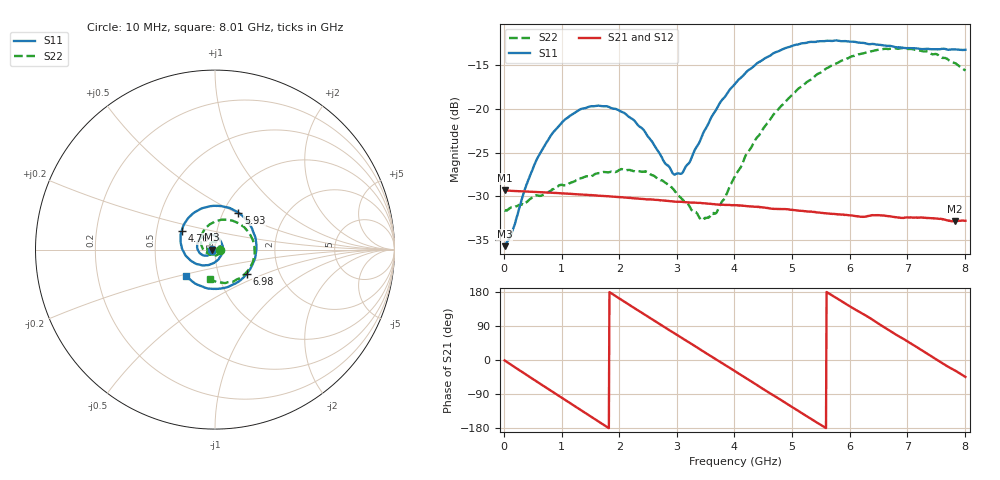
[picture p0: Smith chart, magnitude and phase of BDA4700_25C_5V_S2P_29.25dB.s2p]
!Agilent Technologies,E5071B,MY42404982,A.09.10
!Date: Mon Oct 20 13:41:18 2025
!Data & Calibration Information:
!Freq	S11:SOLT2(ON)	S21:SOLT2(ON)	S12:SOLT2(ON)	S22:SOLT2(ON)
# Hz S RI R 50
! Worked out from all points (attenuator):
!   801 points, 10 MHz to 8.01 GHz, reference 50 ohm
!   highest |S21| = -29.31 dB at 10 MHz (marker M1); lowest = -32.9 dB at 7.83 GHz (marker M2)
!   lowest |S11| = -35.7 dB at 10 MHz (marker M3), VSWR 1.03, Z = 48.4 - j0.111 ohm
!   |S11| at or under -10 dB: start of sweep to end of sweep
!   |S22| runs from -32.7 to -13.0 dB; largest |S21 - S12| = 0.00027
!   S11 on the Smith chart (normalised r, x): 10 MHz: 0.97, -0.00; 4.76 GHz: 0.67, +0.15; 5.93 GHz: 1.18, +0.52; 6.98 GHz: 1.37, -0.38; 8.01 GHz: 0.70, -0.21
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1e7  -0.0164 -0.00114  0.0342 -0.000707  0.0342 -0.000769  0.0262 -0.000817
1.4e8  -0.0175 -0.00941  0.0329 -0.00841  0.033 -0.0084  0.0266 -0.00676
3.8e8  -0.0264 -0.0246  0.0265 -0.0208  0.0265 -0.0209  0.0214 -0.0197
6.2e8  -0.0437 -0.0337  0.0157 -0.0295  0.0157 -0.0295  0.0115 -0.0296
1.01e9  -0.0807 -0.0233  -0.00601 -0.0323  -0.00605 -0.0324  -0.0152 -0.0335
1.35e9  -0.0996 0.01  -0.0225 -0.0233  -0.0225 -0.0233  -0.036 -0.0179
2.08e9  -0.0463 0.0829  -0.0282 0.0133  -0.0282 0.0133  -0.0299 0.0334
2.68e9  0.0318 0.0473  -0.00367 0.0299  -0.00365 0.0299  0.0126 0.0375
2.94e9  0.042 0.00646  0.00901 0.0281  0.0091 0.0281  0.025 0.0243
3.07e9  0.0396 -0.0156  0.0148 0.0254  0.0147 0.0255  0.0277 0.0142
3.44e9  -0.000738 -0.0705  0.0263 0.012  0.0263 0.012  0.0186 -0.0138
3.69e9  -0.0486 -0.0872  0.0284 0.000399  0.0284 0.00036  0.000714 -0.0255
4.01e9  -0.1187 -0.0719  0.0245 -0.0139  0.0245 -0.0139  -0.032 -0.0257
4.76e9  -0.1865 0.1035  -0.00512 -0.0263  -0.00509 -0.0263  -0.0787 0.0605
5.35e9  -0.0626 0.233  -0.0238 -0.01  -0.0238 -0.0101  -0.0156 0.1476
5.93e9  0.13 0.2061  -0.0211 0.0129  -0.0211 0.0129  0.1139 0.1542
6.37e9  0.2203 0.0803  -0.00801 0.0233  -0.00804 0.0231  0.197 0.0806
6.68e9  0.2266 -0.0338  0.00479 0.0239  0.00483 0.024  0.2198 0.000742
6.98e9  0.1778 -0.1335  0.0149 0.0187  0.015 0.0187  0.206 -0.0797
7.41e9  0.0418 -0.2152  0.0233 0.00444  0.0234 0.00441  0.1264 -0.164
7.83e9  -0.111 -0.1888  0.0201 -0.0106  0.0202 -0.0107  0.0137 -0.1819
8.01e9  -0.1617 -0.1454  0.0163 -0.0161  0.0163 -0.0162  -0.0301 -0.1625
